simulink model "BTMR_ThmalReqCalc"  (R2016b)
settings: Solver=FixedStepDiscrete  StartTime=0.0  StopTime=10.0  FixedStep=0.1  RelTol=1e-3  EnableMultiTasking=on
undefined symbols (not defined in the file or in its folder): BMS_cntThmStbNum_C, BTMR_cntThmalReqVal_C, BTMR_flgCoolPwrCal_C, BTMR_pChrgClntPwrLv1_C, BTMR_pChrgClntPwrLv2_C, BTMR_pChrgClntPwrLv3_C, BTMR_pChrgClntPwrLv4_C, BTMR_pChrgClntPwrLv5_C, BTMR_pChrgClntPwrLv6_C, BTMR_pCoolPwrVal_C, BTMR_pHtgACPwrReq_C, BTMR_pHtgDCPwrReq_C, BTMR_pHtgDrvPwrReq_C, BTMR_pHtgsStage1_CUR, BTMR_pHtgsStage2_CUR, BTMR_pNormClntPwrLv1_C, BTMR_pNormClntPwrLv2_C, BTMR_pNormClntPwrLv3_C, BTMR_r861BrsDrvSoc_C, BTMR_r861HtgDrvSoc_C, BTMR_r891BrsDrvSoc_C, BTMR_r891HtgDrvSoc_C, BTMR_rCoolClbFlg_C, BTMR_rFlashClbFlg_C, BTMR_rHeatClbFlg_C, BTMR_t861BrsDiffLv0Temp_C, BTMR_t861BrsDiffLv1Temp_C, BTMR_t861CoolChrgAces2Temp_C, BTMR_t861CoolChrgAces3Temp_C, BTMR_t861CoolChrgAcesTemp_C, BTMR_t861CoolChrgDiffDebTemp_C, BTMR_t861CoolChrgEndDiffTemp_C, BTMR_t861CoolChrgExitLv2Temp_C, BTMR_t861CoolChrgExitLv3Temp_C, BTMR_t861CoolChrgExitTemp_C, BTMR_t861CoolChrgIntLv0Temp_C, BTMR_t861CoolChrgIntLv1Temp_C, BTMR_t861CoolChrgIntLv2Temp_C, BTMR_t861CoolChrgIntLv3Temp_C, BTMR_t861CoolChrgIntLv4Temp_C, BTMR_t861CoolChrgIntLv5Temp_C, BTMR_t861CoolDCDebTemp_C, BTMR_t861CoolNormAcesTemp_C, BTMR_t861CoolNormDiffDebTemp_C, BTMR_t861CoolNormEndDiffTemp_C, BTMR_t861CoolNormExitLv2Temp_C, BTMR_t861CoolNormExitLv3Temp_C, BTMR_t861CoolNormExitTemp_C, BTMR_t861CoolNormIntLv0Temp_C, BTMR_t861CoolNormIntLv1Temp_C, BTMR_t861CoolNormLv2Temp_C, BTMR_t861CoolNormLv3Temp_C, BTMR_t861HtgACDiffDebTemp_C, BTMR_t861HtgACEndDiffTemp_C, BTMR_t861HtgACStartHiTemp_C, BTMR_t861HtgACStartLoTemp_C, BTMR_t861HtgACStopTemp_C, BTMR_t861HtgDCDiffDebTemp_C, BTMR_t861HtgDCEndDiffTemp_C, BTMR_t861HtgDCIntLv0Temp_C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
libraries: AIWAYS_Powertrain_BMS_lib x78, simulink x9
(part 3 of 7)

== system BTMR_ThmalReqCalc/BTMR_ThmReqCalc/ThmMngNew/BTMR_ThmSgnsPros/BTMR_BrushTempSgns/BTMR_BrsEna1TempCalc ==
  BSPR_tCellTempMin : Inport
  BSPR_tCellTempMax : Inport  Port=2
  BMSDebounceStartZero : AIWAYS_Powertrain_BMS_lib/Debounce & Delay/BMSDebounceStartZero
  Constant1 : Constant  Value=BTMR_tiTempBase_C
  Constant13 : Constant  Value=BTMR_t891CoolChrgAcesTemp_C
  Constant17 : Constant  Value=BTMR_t891HtgDCStartHiTemp_C
  Constant2 : Constant  Value=BTMR_tiTempDebs_C
  Logical Operator2 : Logic  AllPortsSameDT=off  OutDataTypeStr=boolean
  Relational Operator8 : RelationalOperator  OutDataTypeStr=boolean  RndMeth=Simplest
  Relational Operator9 : RelationalOperator  Operator=<  OutDataTypeStr=boolean  RndMeth=Simplest
  BTMR_flgBrsEna1Temp : Outport
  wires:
  Relational Operator8/1 -> Logical Operator2/1
  Relational Operator9/1 -> Logical Operator2/2
  Constant13/1 -> Relational Operator9/2
  Constant17/1 -> Relational Operator8/2
  BSPR_tCellTempMin/1 -> Relational Operator8/1
  BSPR_tCellTempMax/1 -> Relational Operator9/1
  Logical Operator2/1 -> BMSDebounceStartZero/1
  BMSDebounceStartZero/1 -> BTMR_flgBrsEna1Temp/1
  Constant2/1 -> BMSDebounceStartZero/4, BMSDebounceStartZero/2
  Constant1/1 -> BMSDebounceStartZero/5, BMSDebounceStartZero/3

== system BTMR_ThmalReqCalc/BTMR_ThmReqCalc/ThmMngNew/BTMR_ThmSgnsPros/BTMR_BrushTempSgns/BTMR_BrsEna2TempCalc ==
  BSPR_tCellTempMin : Inport
  BSPR_tCellTempMax : Inport  Port=2
  BMSDebounceStartZero : AIWAYS_Powertrain_BMS_lib/Debounce & Delay/BMSDebounceStartZero
  Constant1 : Constant  Value=BTMR_tiTempBase_C
  Constant14 : Constant  Value=BTMR_t891HtgACStartHiTemp_C
  Constant16 : Constant  Value=BTMR_t891CoolNormAcesTemp_C
  Constant2 : Constant  Value=BTMR_tiTempDebs_C
  Logical Operator3 : Logic  AllPortsSameDT=off  OutDataTypeStr=boolean
  Relational Operator10 : RelationalOperator  OutDataTypeStr=boolean  RndMeth=Simplest
  Relational Operator11 : RelationalOperator  Operator=<  OutDataTypeStr=boolean  RndMeth=Simplest
  BTMR_flgBrsEna2Temp : Outport
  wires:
  BMSDebounceStartZero/1 -> BTMR_flgBrsEna2Temp/1
  BSPR_tCellTempMax/1 -> Relational Operator11/1
  BSPR_tCellTempMin/1 -> Relational Operator10/1
  Logical Operator3/1 -> BMSDebounceStartZero/1
  Relational Operator10/1 -> Logical Operator3/1
  Relational Operator11/1 -> Logical Operator3/2
  Constant14/1 -> Relational Operator10/2
  Constant16/1 -> Relational Operator11/2
  Constant2/1 -> BMSDebounceStartZero/4, BMSDebounceStartZero/2
  Constant1/1 -> BMSDebounceStartZero/5, BMSDebounceStartZero/3

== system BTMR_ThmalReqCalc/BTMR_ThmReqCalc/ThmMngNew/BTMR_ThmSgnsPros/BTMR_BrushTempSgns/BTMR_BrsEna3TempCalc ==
  BSPR_tCellTempMin : Inport
  BSPR_tCellTempMax : Inport  Port=2
  BMSDebounceStartZero : AIWAYS_Powertrain_BMS_lib/Debounce & Delay/BMSDebounceStartZero
  Constant1 : Constant  Value=BTMR_tiTempBase_C
  Constant19 : Constant  Value=BTMR_t891CoolNormAcesTemp_C
  Constant2 : Constant  Value=BTMR_tiTempDebs_C
  Constant20 : Constant  Value=BTMR_t891HtgDrvStartHiTemp_C
  Logical Operator4 : Logic  AllPortsSameDT=off  OutDataTypeStr=boolean
  Relational Operator12 : RelationalOperator  Operator=>  OutDataTypeStr=boolean  RndMeth=Simplest
  Relational Operator13 : RelationalOperator  Operator=<  OutDataTypeStr=boolean  RndMeth=Simplest
  BTMR_flgBrsEna3Temp : Outport
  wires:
  BSPR_tCellTempMax/1 -> Relational Operator13/1
  BMSDebounceStartZero/1 -> BTMR_flgBrsEna3Temp/1
  Relational Operator12/1 -> Logical Operator4/1
  Constant19/1 -> Relational Operator13/2
  Relational Operator13/1 -> Logical Operator4/2
  Constant20/1 -> Relational Operator12/2
  Logical Operator4/1 -> BMSDebounceStartZero/1
  BSPR_tCellTempMin/1 -> Relational Operator12/1
  Constant2/1 -> BMSDebounceStartZero/4, BMSDebounceStartZero/2
  Constant1/1 -> BMSDebounceStartZero/5, BMSDebounceStartZero/3

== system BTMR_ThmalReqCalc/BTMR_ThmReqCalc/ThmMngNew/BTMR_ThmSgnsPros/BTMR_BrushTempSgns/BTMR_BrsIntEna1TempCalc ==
  BSPR_tClntUsT : Inport
  BMSDebounceStartZero : AIWAYS_Powertrain_BMS_lib/Debounce & Delay/BMSDebounceStartZero
  Constant1 : Constant  Value=BTMR_tiTempBase_C
  Constant13 : Constant  Value=BTMR_t891CoolChrgAcesTemp_C
  Constant17 : Constant  Value=BTMR_t891HtgDCStartHiTemp_C
  Constant2 : Constant  Value=BTMR_tiTempDebs_C
  Logical Operator2 : Logic  AllPortsSameDT=off  OutDataTypeStr=boolean
  Relational Operator8 : RelationalOperator  OutDataTypeStr=boolean  RndMeth=Simplest
  Relational Operator9 : RelationalOperator  Operator=<  OutDataTypeStr=boolean  RndMeth=Simplest
  BTMR_flgBrsIntEna1Temp : Outport
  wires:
  BMSDebounceStartZero/1 -> BTMR_flgBrsIntEna1Temp/1
  Logical Operator2/1 -> BMSDebounceStartZero/1
  BSPR_tClntUsT/1 -> Relational Operator9/1, Relational Operator8/1
  Constant17/1 -> Relational Operator8/2
  Constant13/1 -> Relational Operator9/2
  Relational Operator9/1 -> Logical Operator2/2
  Relational Operator8/1 -> Logical Operator2/1
  Constant2/1 -> BMSDebounceStartZero/4, BMSDebounceStartZero/2
  Constant1/1 -> BMSDebounceStartZero/5, BMSDebounceStartZero/3

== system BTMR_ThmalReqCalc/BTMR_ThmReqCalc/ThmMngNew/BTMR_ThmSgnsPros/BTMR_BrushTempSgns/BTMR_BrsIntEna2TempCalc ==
  BSPR_tClntUsT : Inport
  BMSDebounceStartZero : AIWAYS_Powertrain_BMS_lib/Debounce & Delay/BMSDebounceStartZero
  Constant1 : Constant  Value=BTMR_tiTempBase_C
  Constant14 : Constant  Value=BTMR_t891HtgACStartHiTemp_C
  Constant16 : Constant  Value=BTMR_t891CoolNormAcesTemp_C
  Constant2 : Constant  Value=BTMR_tiTempDebs_C
  Logical Operator3 : Logic  AllPortsSameDT=off  OutDataTypeStr=boolean
  Relational Operator10 : RelationalOperator  OutDataTypeStr=boolean  RndMeth=Simplest
  Relational Operator11 : RelationalOperator  Operator=<  OutDataTypeStr=boolean  RndMeth=Simplest
  BTMR_flgBrsIntEna2Temp : Outport
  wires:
  Constant16/1 -> Relational Operator11/2
  Constant14/1 -> Relational Operator10/2
  Relational Operator11/1 -> Logical Operator3/2
  Relational Operator10/1 -> Logical Operator3/1
  Logical Operator3/1 -> BMSDebounceStartZero/1
  BSPR_tClntUsT/1 -> Relational Operator11/1, Relational Operator10/1
  BMSDebounceStartZero/1 -> BTMR_flgBrsIntEna2Temp/1
  Constant2/1 -> BMSDebounceStartZero/4, BMSDebounceStartZero/2
  Constant1/1 -> BMSDebounceStartZero/5, BMSDebounceStartZero/3

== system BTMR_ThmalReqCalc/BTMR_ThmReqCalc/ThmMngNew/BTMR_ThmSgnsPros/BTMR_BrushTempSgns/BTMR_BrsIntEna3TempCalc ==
  BSPR_tClntUsT : Inport
  BMSDebounceStartZero : AIWAYS_Powertrain_BMS_lib/Debounce & Delay/BMSDebounceStartZero
  Constant1 : Constant  Value=BTMR_tiTempBase_C
  Constant19 : Constant  Value=BTMR_t891CoolNormAcesTemp_C
  Constant2 : Constant  Value=BTMR_tiTempDebs_C
  Constant20 : Constant  Value=BTMR_t891HtgDrvStartHiTemp_C
  Logical Operator4 : Logic  AllPortsSameDT=off  OutDataTypeStr=boolean
  Relational Operator12 : RelationalOperator  Operator=>  OutDataTypeStr=boolean  RndMeth=Simplest
  Relational Operator13 : RelationalOperator  Operator=<  OutDataTypeStr=boolean  RndMeth=Simplest
  BTMR_flgBrsIntEna3Temp : Outport
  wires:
  Logical Operator4/1 -> BMSDebounceStartZero/1
  Constant20/1 -> Relational Operator12/2
  Relational Operator13/1 -> Logical Operator4/2
  Constant19/1 -> Relational Operator13/2
  Relational Operator12/1 -> Logical Operator4/1
  BMSDebounceStartZero/1 -> BTMR_flgBrsIntEna3Temp/1
  BSPR_tClntUsT/1 -> Relational Operator13/1, Relational Operator12/1
  Constant2/1 -> BMSDebounceStartZero/4, BMSDebounceStartZero/2
  Constant1/1 -> BMSDebounceStartZero/5, BMSDebounceStartZero/3

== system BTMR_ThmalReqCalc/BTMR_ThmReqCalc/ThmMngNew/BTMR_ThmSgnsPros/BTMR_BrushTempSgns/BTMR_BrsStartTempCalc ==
  BSPR_tCellTempMin : Inport
  BSPR_tCellTempMax : Inport  Port=2
  Add : Sum  Inputs=+-
  BMSDebounceStartZero : AIWAYS_Powertrain_BMS_lib/Debounce & Delay/BMSDebounceStartZero
  Constant1 : Constant  Value=BTMR_tiTempBase_C
  Constant2 : Constant  Value=BTMR_t891BrsDiffLv1Temp_C
  Constant3 : Constant  Value=BTMR_tiTempDebs_C
  Constant4 : Constant  Value=BTMR_tBrsMinCellTempThre_C
  Logical Operator4 : Logic  AllPortsSameDT=off  OutDataTypeStr=boolean
  Relational Operator2 : RelationalOperator  OutDataTypeStr=boolean  RndMeth=Simplest
  Relational Operator4 : RelationalOperator  OutDataTypeStr=boolean  RndMeth=Simplest
  BTMR_flgBrsStartTemp : Outport
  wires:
  BMSDebounceStartZero/1 -> BTMR_flgBrsStartTemp/1
  Add/1 -> Relational Operator2/1
  Constant2/1 -> Relational Operator2/2
  Relational Operator2/1 -> Logical Operator4/1
  BSPR_tCellTempMax/1 -> Add/1
  Constant3/1 -> BMSDebounceStartZero/4, BMSDebounceStartZero/2
  Constant1/1 -> BMSDebounceStartZero/5, BMSDebounceStartZero/3
  BSPR_tCellTempMin/1 -> Relational Operator4/1, Add/2
  Constant4/1 -> Relational Operator4/2
  Relational Operator4/1 -> Logical Operator4/2
  Logical Operator4/1 -> BMSDebounceStartZero/1

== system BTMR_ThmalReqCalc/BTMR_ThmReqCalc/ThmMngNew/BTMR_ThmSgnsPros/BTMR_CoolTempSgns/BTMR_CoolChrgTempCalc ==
  BSPR_tCellTempMax : Inport
  BTMR_CoolChrgDnaTempCalc : Subsystem
  BTMR_CoolChrgStage2EnaTempCalc : Subsystem
  BTMR_CoolChrgStage2ExtTempCalc : Subsystem
  BTMR_CoolChrgStage3EnaTempCalc : Subsystem
  BTMR_CoolChrgStage3ExtTempCalc : Subsystem
  Bus Creator : BusCreator  Inputs=5
  BTMR_flgCoolChrgTempSgns : Outport
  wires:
  BTMR_CoolChrgStage2EnaTempCalc/1(BTMR_flgCoolChrgStage2EnaTemp) -> Bus Creator/2  "BTMR_flgCoolChrgStage2EnaTemp"
  BTMR_CoolChrgStage3EnaTempCalc/1(BTMR_flgCoolChrgStage3EnaTemp) -> Bus Creator/3  "BTMR_flgCoolChrgStage3EnaTemp"
  BTMR_CoolChrgStage3ExtTempCalc/1(BTMR_flgCoolChrgStage3ExtTemp) -> Bus Creator/5  "BTMR_flgCoolChrgStage3ExtTemp"
  BTMR_CoolChrgStage2ExtTempCalc/1(BTMR_flgCoolChrgStage2ExtTemp) -> Bus Creator/4  "BTMR_flgCoolChrgStage2ExtTemp"
  BSPR_tCellTempMax/1 -> BTMR_CoolChrgStage3ExtTempCalc/1(BSPR_tCellTempMax), BTMR_CoolChrgStage2ExtTempCalc/1(BSPR_tCellTempMax), BTMR_CoolChrgDnaTempCalc/1(BSPR_tCellTempMax), BTMR_CoolChrgStage2EnaTempCalc/1(BSPR_tCellTempMax), BTMR_CoolChrgStage3EnaTempCalc/1(BSPR_tCellTempMax)
  BTMR_CoolChrgDnaTempCalc/1(BTMR_flgCoolChrgDnaTemp) -> Bus Creator/1  "BTMR_flgCoolChrgDnaTemp"
  Bus Creator/1 -> BTMR_flgCoolChrgTempSgns/1  "BTMR_flgCoolChrgTempSgns"

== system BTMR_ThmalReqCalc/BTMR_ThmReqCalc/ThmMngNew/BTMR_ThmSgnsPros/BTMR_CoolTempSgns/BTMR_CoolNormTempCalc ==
  BSPR_tCellTempMax : Inport
  BTMR_CoolNormDnaTempCalc : Subsystem
  BTMR_CoolNormStage2EnaTempCalc : Subsystem
  BTMR_CoolNormStage2ExtTempCalc : Subsystem
  BTMR_CoolNormStage3EnaTempCalc : Subsystem
  BTMR_CoolNormStage3ExtTempCalc : Subsystem
  Bus Creator : BusCreator  Inputs=5
  BTMR_flgCoolNormTempSgns : Outport
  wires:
  BTMR_CoolNormDnaTempCalc/1(BTMR_flgCoolNormDnaTemp) -> Bus Creator/1  "BTMR_flgCoolNormDnaTemp"
  BTMR_CoolNormStage2EnaTempCalc/1(BTMR_flgCoolNormStage2EnaTemp) -> Bus Creator/2  "BTMR_flgCoolNormStage2EnaTemp"
  BTMR_CoolNormStage3EnaTempCalc/1(BTMR_flgCoolNormStage3EnaTemp) -> Bus Creator/3  "BTMR_flgCoolNormStage3EnaTemp"
  BTMR_CoolNormStage3ExtTempCalc/1(BTMR_flgCoolNormStage3ExtTemp) -> Bus Creator/5  "BTMR_flgCoolNormStage3ExtTemp"
  BTMR_CoolNormStage2ExtTempCalc/1(BTMR_flgCoolNormStage2ExtTemp) -> Bus Creator/4  "BTMR_flgCoolNormStage2ExtTemp"
  BSPR_tCellTempMax/1 -> BTMR_CoolNormDnaTempCalc/1(BSPR_tCellTempMax), BTMR_CoolNormStage2EnaTempCalc/1(BSPR_tCellTempMax), BTMR_CoolNormStage3ExtTempCalc/1(BSPR_tCellTempMax), BTMR_CoolNormStage2ExtTempCalc/1(BSPR_tCellTempMax), BTMR_CoolNormStage3EnaTempCalc/1(BSPR_tCellTempMax)
  Bus Creator/1 -> BTMR_flgCoolNormTempSgns/1  "BTMR_flgCoolNormTempSgns"

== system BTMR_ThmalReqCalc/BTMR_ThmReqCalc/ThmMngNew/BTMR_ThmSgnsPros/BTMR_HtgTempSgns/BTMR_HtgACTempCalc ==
  BSPR_tCellTempMin : Inport
  BSPR_tCellTempMax : Inport  Port=2
  BTMR_HtgACDnaTempCalc : Subsystem
  Bus Creator : BusCreator  Inputs=1
  BTMR_flgHtgACTempSgns : Outport
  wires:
  BTMR_HtgACDnaTempCalc/1(BTMR_flgHtgACDnaTemp) -> Bus Creator/1  "BTMR_flgHtgACDnaTemp"
  BSPR_tCellTempMin/1 -> BTMR_HtgACDnaTempCalc/1(BSPR_tCellTempMin)
  Bus Creator/1 -> BTMR_flgHtgACTempSgns/1  "BTMR_flgHtgACTempSgns"
  BSPR_tCellTempMax/1 -> BTMR_HtgACDnaTempCalc/2(BSPR_tCellTempMax)

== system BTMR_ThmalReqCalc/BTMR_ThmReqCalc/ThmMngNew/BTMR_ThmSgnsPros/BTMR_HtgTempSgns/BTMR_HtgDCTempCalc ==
  BSPR_tCellTempMin : Inport
  BSPR_tCellTempMax : Inport  Port=2
  BTMR_HtgDCDnaTempCalc : Subsystem
  BTMR_HtgDCStage2EnaTempCalc : Subsystem
  Bus Creator : BusCreator  Inputs=2
  BTMR_flgHtgDCTempSgns : Outport
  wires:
  BSPR_tCellTempMax/1 -> BTMR_HtgDCDnaTempCalc/2(BSPR_tCellTempMax), BTMR_HtgDCStage2EnaTempCalc/2(BSPR_tCellTempMax)
  BTMR_HtgDCDnaTempCalc/1(BTMR_flgHtgDCDnaTemp) -> Bus Creator/2  "BTMR_flgHtgDCDnaTemp"
  BTMR_HtgDCStage2EnaTempCalc/1(BTMR_flgHtgDCStage2EnaTemp) -> Bus Creator/1  "BTMR_flgHtgDCStage2EnaTemp"
  BSPR_tCellTempMin/1 -> BTMR_HtgDCDnaTempCalc/1(BSPR_tCellTempMin), BTMR_HtgDCStage2EnaTempCalc/1(BSPR_tCellTempMin)
  Bus Creator/1 -> BTMR_flgHtgDCTempSgns/1  "BTMR_flgHtgDCTempSgns"

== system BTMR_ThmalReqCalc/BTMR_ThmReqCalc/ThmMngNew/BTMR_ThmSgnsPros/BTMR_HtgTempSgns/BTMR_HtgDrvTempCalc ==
  BSPR_tCellTempMin : Inport
  BSPR_tCellTempMax : Inport  Port=2
  BTMR_HtgDrvDnaTempCalc : Subsystem
  Bus Creator : BusCreator  Inputs=1
  BTMR_flgHtgDrvTempSgns : Outport
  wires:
  BTMR_HtgDrvDnaTempCalc/1(BTMR_flgHtgDrvDnaTemp) -> Bus Creator/1  "BTMR_flgHtgDrvDnaTemp"
  BSPR_tCellTempMin/1 -> BTMR_HtgDrvDnaTempCalc/1(BSPR_tCellTempMin)
  Bus Creator/1 -> BTMR_flgHtgDrvTempSgns/1  "BTMR_flgHtgDrvTempSgns"
  BSPR_tCellTempMax/1 -> BTMR_HtgDrvDnaTempCalc/2(BSPR_tCellTempMax)

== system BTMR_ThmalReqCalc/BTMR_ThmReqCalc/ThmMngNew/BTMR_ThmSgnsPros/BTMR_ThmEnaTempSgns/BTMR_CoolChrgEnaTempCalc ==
  BSPR_tCellTempMin : Inport
  BSPR_tCellTempMax : Inport  Port=2
  Add : Sum
  Add1 : Sum  Inputs=+-
  Add2 : Sum  Inputs=+-
  BMSDebounceStartZero : AIWAYS_Powertrain_BMS_lib/Debounce & Delay/BMSDebounceStartZero
  Constant1 : Constant  Value=BTMR_tiTempBase_C
  Constant2 : Constant  Value=BTMR_tiTempDebs_C
  Constant27 : Constant  Value=BTMR_t891CoolChrgAcesTemp_C
  Constant3 : Constant  Value=BTMR_t891HtgDCStopMinTemp_C
  Constant4 : Constant  Value=BTMR_t891CoolDCDebTemp_C
  Constant5 : Constant  Value=BTMR_t891CoolChrgDiffDebTemp_C
  Constant6 : Constant  Value=BTMR_t891CoolChrgEndDiffTemp_C
  Logical Operator : Logic  Inputs=3  AllPortsSameDT=off  OutDataTypeStr=boolean
  Relational Operator1 : RelationalOperator  OutDataTypeStr=boolean  RndMeth=Simplest
  Relational Operator19 : RelationalOperator  OutDataTypeStr=boolean  RndMeth=Simplest
  Relational Operator2 : RelationalOperator  Operator=<  OutDataTypeStr=boolean  RndMeth=Simplest
  BTMR_flgCoolChrgEnaTemp : Outport
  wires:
  Logical Operator/1 -> BMSDebounceStartZero/1
  Constant27/1 -> Relational Operator19/2
  BMSDebounceStartZero/1 -> BTMR_flgCoolChrgEnaTemp/1
  Constant2/1 -> BMSDebounceStartZero/4, BMSDebounceStartZero/2
  Constant1/1 -> BMSDebounceStartZero/5, BMSDebounceStartZero/3
  Add1/1 -> Relational Operator2/1
  Relational Operator1/1 -> Logical Operator/3
  Add2/1 -> Relational Operator2/2
  Add/1 -> Relational Operator1/2
  Constant5/1 -> Add2/2
  BSPR_tCellTempMax/1 -> Add1/1, Relational Operator19/1
  BSPR_tCellTempMin/1 -> Relational Operator1/1, Add1/2
  Relational Operator2/1 -> Logical Operator/2
  Constant4/1 -> Add/2
  Constant3/1 -> Add/1
  Constant6/1 -> Add2/1
  Relational Operator19/1 -> Logical Operator/1

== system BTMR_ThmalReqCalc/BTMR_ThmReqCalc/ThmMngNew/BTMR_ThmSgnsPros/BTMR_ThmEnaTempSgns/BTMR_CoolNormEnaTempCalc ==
  BSPR_tCellTempMin : Inport
  BSPR_tCellTempMax : Inport  Port=2
  Add1 : Sum  Inputs=+-
  Add2 : Sum  Inputs=+-
  BMSDebounceStartZero : AIWAYS_Powertrain_BMS_lib/Debounce & Delay/BMSDebounceStartZero
  Constant1 : Constant  Value=BTMR_tiTempBase_C
  Constant2 : Constant  Value=BTMR_tiTempDebs_C
  Constant28 : Constant  Value=BTMR_t891CoolNormAcesTemp_C
  Constant3 : Constant  Value=BTMR_t891CoolNormDiffDebTemp_C
  Constant4 : Constant  Value=BTMR_t891CoolNormEndDiffTemp_C
  Logical Operator : Logic  AllPortsSameDT=off  OutDataTypeStr=boolean
  Relational Operator2 : RelationalOperator  Operator=<  OutDataTypeStr=boolean  RndMeth=Simplest
  Relational Operator20 : RelationalOperator  OutDataTypeStr=boolean  RndMeth=Simplest
  BTMR_flgCoolNormEnaTemp : Outport
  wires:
  Logical Operator/1 -> BMSDebounceStartZero/1
  BMSDebounceStartZero/1 -> BTMR_flgCoolNormEnaTemp/1
  Constant28/1 -> Relational Operator20/2
  Constant2/1 -> BMSDebounceStartZero/4, BMSDebounceStartZero/2
  Constant1/1 -> BMSDebounceStartZero/5, BMSDebounceStartZero/3
  Add2/1 -> Relational Operator2/2
  BSPR_tCellTempMin/1 -> Add1/2
  Constant3/1 -> Add2/2
  Add1/1 -> Relational Operator2/1
  Constant4/1 -> Add2/1
  BSPR_tCellTempMax/1 -> Add1/1, Relational Operator20/1
  Relational Operator20/1 -> Logical Operator/1
  Relational Operator2/1 -> Logical Operator/2

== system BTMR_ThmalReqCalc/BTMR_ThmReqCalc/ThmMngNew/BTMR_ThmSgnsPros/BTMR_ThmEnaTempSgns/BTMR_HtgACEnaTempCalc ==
  BSPR_tCellTempMin : Inport
  BSPR_tCellTempMax : Inport  Port=2
  BMSDebounceStartZero : AIWAYS_Powertrain_BMS_lib/Debounce & Delay/BMSDebounceStartZero
  Constant1 : Constant  Value=BTMR_tiTempBase_C
  Constant2 : Constant  Value=BTMR_tiTempDebs_C
  Constant23 : Constant  Value=BTMR_t891HtgACStartLoTemp_C
  Constant24 : Constant  Value=BTMR_t891HtgACStartHiTemp_C
  Constant3 : Constant  Value=BTMR_t891HtgACDiffDebTemp_C
  Constant4 : Constant  Value=BTMR_t891HtgACEndDiffTemp_C
  Logical Operator6 : Logic  Inputs=3  AllPortsSameDT=off  OutDataTypeStr=boolean
  Relational Operator1 : RelationalOperator  Operator=<  OutDataTypeStr=boolean  RndMeth=Simplest
  Relational Operator14 : RelationalOperator  OutDataTypeStr=boolean  RndMeth=Simplest
  Relational Operator15 : RelationalOperator  Operator=<  OutDataTypeStr=boolean  RndMeth=Simplest
  Sum1 : Sum  Inputs=+-  OutDataTypeStr=Inherit: Inherit via back propagation  RndMeth=Zero
  Sum2 : Sum  Inputs=+-  OutDataTypeStr=Inherit: Inherit via back propagation  RndMeth=Zero
  BTMR_flgHtgACEnaTemp : Outport
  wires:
  BMSDebounceStartZero/1 -> BTMR_flgHtgACEnaTemp/1
  Relational Operator14/1 -> Logical Operator6/2
  Constant24/1 -> Relational Operator15/2
  Constant23/1 -> Relational Operator14/2
  Relational Operator15/1 -> Logical Operator6/3
  Logical Operator6/1 -> BMSDebounceStartZero/1
  Constant2/1 -> BMSDebounceStartZero/4, BMSDebounceStartZero/2
  Constant1/1 -> BMSDebounceStartZero/5, BMSDebounceStartZero/3
  Constant3/1 -> Sum2/2
  Sum2/1 -> Relational Operator1/2
  BSPR_tCellTempMax/1 -> Sum1/1
  Relational Operator1/1 -> Logical Operator6/1
  Sum1/1 -> Relational Operator1/1
  BSPR_tCellTempMin/1 -> Sum1/2, Relational Operator15/1, Relational Operator14/1
  Constant4/1 -> Sum2/1

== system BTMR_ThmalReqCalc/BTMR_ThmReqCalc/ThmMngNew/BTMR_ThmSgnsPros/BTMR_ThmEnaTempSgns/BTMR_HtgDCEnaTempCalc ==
  BSPR_tCellTempMin : Inport
  BSPR_tCellTempMax : Inport  Port=2
  BMSDebounceStartZero : AIWAYS_Powertrain_BMS_lib/Debounce & Delay/BMSDebounceStartZero
  Constant1 : Constant  Value=BTMR_tiTempBase_C
  Constant2 : Constant  Value=BTMR_tiTempDebs_C
  Constant23 : Constant  Value=BTMR_t891HtgDCStopMaxTemp_C
  Constant25 : Constant  Value=BTMR_t891HtgDCStartHiTemp_C
  Constant26 : Constant  Value=BTMR_t891HtgDCStartLoTemp_C
  Constant3 : Constant  Value=BTMR_t891HtgDCDiffDebTemp_C
  Constant4 : Constant  Value=BTMR_t891HtgDCEndDiffTemp_C
  Constant5 : Constant  Value=BTMR_tHtgDCMaxTempDeb_C
  Logical Operator6 : Logic  Inputs=4  AllPortsSameDT=off  OutDataTypeStr=boolean
  Relational Operator1 : RelationalOperator  Operator=<  OutDataTypeStr=boolean  RndMeth=Simplest
  Relational Operator16 : RelationalOperator  Operator=>  OutDataTypeStr=boolean  RndMeth=Simplest
  Relational Operator17 : RelationalOperator  Operator=<  OutDataTypeStr=boolean  RndMeth=Simplest
  Relational Operator2 : RelationalOperator  Operator=<  OutDataTypeStr=boolean  RndMeth=Simplest
  Sum1 : Sum  Inputs=+-  OutDataTypeStr=Inherit: Inherit via back propagation  RndMeth=Zero
  Sum2 : Sum  Inputs=+-  OutDataTypeStr=Inherit: Inherit via back propagation  RndMeth=Zero
  Sum3 : Sum  Inputs=+-  OutDataTypeStr=Inherit: Inherit via back propagation  RndMeth=Zero
  BTMR_flgHtgDCEnaTemp : Outport
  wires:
  BMSDebounceStartZero/1 -> BTMR_flgHtgDCEnaTemp/1
  Constant25/1 -> Relational Operator17/2
  Relational Operator17/1 -> Logical Operator6/4
  Constant26/1 -> Relational Operator16/2
  Relational Operator16/1 -> Logical Operator6/3
  Logical Operator6/1 -> BMSDebounceStartZero/1
  Constant2/1 -> BMSDebounceStartZero/4, BMSDebounceStartZero/2
  Constant1/1 -> BMSDebounceStartZero/5, BMSDebounceStartZero/3
  Sum1/1 -> Relational Operator1/1
  BSPR_tCellTempMin/1 -> Relational Operator17/1, Relational Operator16/1, Sum1/2
  BSPR_tCellTempMax/1 -> Sum1/1, Relational Operator2/1
  Sum2/1 -> Relational Operator1/2
  Constant3/1 -> Sum2/2
  Constant4/1 -> Sum2/1
  Relational Operator1/1 -> Logical Operator6/2
  Constant23/1 -> Sum3/1
  Constant5/1 -> Sum3/2
  Sum3/1 -> Relational Operator2/2
  Relational Operator2/1 -> Logical Operator6/1

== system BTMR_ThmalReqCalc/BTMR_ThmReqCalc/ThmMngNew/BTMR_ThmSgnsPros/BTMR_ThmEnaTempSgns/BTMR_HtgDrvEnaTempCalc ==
  BSPR_tCellTempMin : Inport
  BSPR_tCellTempMax : Inport  Port=2
  BMSDebounceStartZero : AIWAYS_Powertrain_BMS_lib/Debounce & Delay/BMSDebounceStartZero
  Constant1 : Constant  Value=BTMR_tiTempBase_C
  Constant2 : Constant  Value=BTMR_tiTempDebs_C
  Constant21 : Constant  Value=BTMR_t891HtgDrvStartLoTemp_C
  Constant22 : Constant  Value=BTMR_t891HtgDrvStartHiTemp_C
  Constant3 : Constant  Value=BTMR_t891HtgDrvDiffDebTemp_C
  Constant4 : Constant  Value=BTMR_t891HtgDrvEndDiffTemp_C
  Logical Operator6 : Logic  Inputs=3  AllPortsSameDT=off  OutDataTypeStr=boolean
  Relational Operator1 : RelationalOperator  OutDataTypeStr=boolean  RndMeth=Simplest
  Relational Operator18 : RelationalOperator  Operator=<=  OutDataTypeStr=boolean  RndMeth=Simplest
  Relational Operator2 : RelationalOperator  Operator=<  OutDataTypeStr=boolean  RndMeth=Simplest
  Sum1 : Sum  Inputs=+-  OutDataTypeStr=Inherit: Inherit via back propagation  RndMeth=Zero
  Sum2 : Sum  Inputs=+-  OutDataTypeStr=Inherit: Inherit via back propagation  RndMeth=Zero
  BTMR_flgHtgDrvEnaTemp : Outport
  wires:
  Constant22/1 -> Relational Operator18/2
  BMSDebounceStartZero/1 -> BTMR_flgHtgDrvEnaTemp/1
  Logical Operator6/1 -> BMSDebounceStartZero/1
  Constant21/1 -> Relational Operator1/2
  Relational Operator18/1 -> Logical Operator6/2
  Relational Operator1/1 -> Logical Operator6/3
  Constant2/1 -> BMSDebounceStartZero/4, BMSDebounceStartZero/2
  Constant1/1 -> BMSDebounceStartZero/5, BMSDebounceStartZero/3
  Sum1/1 -> Relational Operator2/1
  Constant4/1 -> Sum2/1
  Sum2/1 -> Relational Operator2/2
  BSPR_tCellTempMax/1 -> Sum1/1
  Constant3/1 -> Sum2/2
  Relational Operator2/1 -> Logical Operator6/1
  BSPR_tCellTempMin/1 -> Sum1/2, Relational Operator1/1, Relational Operator18/1

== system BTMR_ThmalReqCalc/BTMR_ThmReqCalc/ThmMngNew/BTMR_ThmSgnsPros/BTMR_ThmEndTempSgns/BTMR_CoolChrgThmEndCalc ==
  BTMR_flgBMSSgns : Inport
  BSPR_tCellTempMax : Inport  Port=2
  BSPR_tCellTempMin : Inport  Port=3
  Add : Sum  Inputs=+-
  BMSDebounceStartZero : AIWAYS_Powertrain_BMS_lib/Debounce & Delay/BMSDebounceStartZero
  Bus Selector : BusSelector  OutputSignals=BTMR_flgBMSDChrg
  Constant1 : Constant  Value=BTMR_tiTempBase_C
  Constant14 : Constant  Value=BTMR_t891CoolChrgEndDiffTemp_C
  Constant2 : Constant  Value=BTMR_tiTempDebs_C
  Logical Operator1 : Logic  AllPortsSameDT=off  OutDataTypeStr=boolean
  Relational Operator3 : RelationalOperator  OutDataTypeStr=boolean  RndMeth=Simplest
  BTMR_CoolChrgThmEnd : Outport
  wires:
  BMSDebounceStartZero/1 -> Logical Operator1/2
  BSPR_tCellTempMin/1 -> Add/2
  Add/1 -> Relational Operator3/1
  Constant14/1 -> Relational Operator3/2
  BSPR_tCellTempMax/1 -> Add/1
  Relational Operator3/1 -> BMSDebounceStartZero/1
  BTMR_flgBMSSgns/1 -> Bus Selector/1
  Bus Selector/1 -> Logical Operator1/1  "<BTMR_flgBMSDChrg>"
  Logical Operator1/1 -> BTMR_CoolChrgThmEnd/1
  Constant2/1 -> BMSDebounceStartZero/4, BMSDebounceStartZero/2
  Constant1/1 -> BMSDebounceStartZero/5, BMSDebounceStartZero/3

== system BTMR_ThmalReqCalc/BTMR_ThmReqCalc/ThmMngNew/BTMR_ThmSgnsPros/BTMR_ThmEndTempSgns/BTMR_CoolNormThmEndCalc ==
  BTMR_flgBMSSgns : Inport
  BSPR_tCellTempMax : Inport  Port=2
  BSPR_tCellTempMin : Inport  Port=3
  Add : Sum  Inputs=+-
  BMSDebounceStartZero : AIWAYS_Powertrain_BMS_lib/Debounce & Delay/BMSDebounceStartZero
  Bus Selector : BusSelector  OutputSignals=BTMR_flgBMSAChrg,BTMR_flgBMSDrv
  Constant1 : Constant  Value=BTMR_tiTempBase_C
  Constant14 : Constant  Value=BTMR_t891CoolNormEndDiffTemp_C
  Constant2 : Constant  Value=BTMR_tiTempDebs_C
  Logical Operator1 : Logic  AllPortsSameDT=off  OutDataTypeStr=boolean
  Logical Operator2 : Logic  Operator=OR  AllPortsSameDT=off  OutDataTypeStr=boolean
  Relational Operator3 : RelationalOperator  OutDataTypeStr=boolean  RndMeth=Simplest
  BTMR_CoolNormThmEnd : Outport
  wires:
  BTMR_flgBMSSgns/1 -> Bus Selector/1
  Relational Operator3/1 -> BMSDebounceStartZero/1
  BSPR_tCellTempMax/1 -> Add/1
  Constant14/1 -> Relational Operator3/2
  Add/1 -> Relational Operator3/1
  BSPR_tCellTempMin/1 -> Add/2
  BMSDebounceStartZero/1 -> Logical Operator1/2
  Bus Selector/1 -> Logical Operator2/1  "<BTMR_flgBMSAChrg>"
  Bus Selector/2 -> Logical Operator2/2  "<BTMR_flgBMSDrv>"
  Logical Operator2/1 -> Logical Operator1/1
  Logical Operator1/1 -> BTMR_CoolNormThmEnd/1
  Constant2/1 -> BMSDebounceStartZero/4, BMSDebounceStartZero/2
  Constant1/1 -> BMSDebounceStartZero/5, BMSDebounceStartZero/3

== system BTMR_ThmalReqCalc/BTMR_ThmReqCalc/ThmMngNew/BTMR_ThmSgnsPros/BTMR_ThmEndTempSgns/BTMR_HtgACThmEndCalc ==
  BTMR_flgBMSSgns : Inport
  BSPR_tCellTempMax : Inport  Port=2
  BSPR_tCellTempMin : Inport  Port=3
  BCMR_bAcChrgHeatFbd : Inport  Port=4
  Add : Sum  Inputs=+-
  BMSDebounceStartZero : AIWAYS_Powertrain_BMS_lib/Debounce & Delay/BMSDebounceStartZero
  Bus Selector : BusSelector  OutputSignals=BTMR_flgBMSAChrg
  Constant1 : Constant  Value=BTMR_tiTempBase_C
  Constant14 : Constant  Value=BTMR_t891HtgACEndDiffTemp_C
  Constant2 : Constant  Value=BTMR_tiTempDebs_C
  Logical Operator1 : Logic  AllPortsSameDT=off  OutDataTypeStr=boolean
  Logical Operator2 : Logic  Operator=OR  AllPortsSameDT=off  OutDataTypeStr=boolean
  Relational Operator3 : RelationalOperator  OutDataTypeStr=boolean  RndMeth=Simplest
  BTMR_HtgACThmEnd : Outport
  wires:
  Logical Operator1/1 -> BTMR_HtgACThmEnd/1
  BSPR_tCellTempMin/1 -> Add/2
  Add/1 -> Relational Operator3/1
  Constant14/1 -> Relational Operator3/2
  BSPR_tCellTempMax/1 -> Add/1
  Relational Operator3/1 -> BMSDebounceStartZero/1
  BTMR_flgBMSSgns/1 -> Bus Selector/1
  Bus Selector/1 -> Logical Operator1/1  "<BTMR_flgBMSAChrg>"
  BMSDebounceStartZero/1 -> Logical Operator2/1
  BCMR_bAcChrgHeatFbd/1 -> Logical Operator2/2
  Logical Operator2/1 -> Logical Operator1/2
  Constant2/1 -> BMSDebounceStartZero/4, BMSDebounceStartZero/2
  Constant1/1 -> BMSDebounceStartZero/5, BMSDebounceStartZero/3

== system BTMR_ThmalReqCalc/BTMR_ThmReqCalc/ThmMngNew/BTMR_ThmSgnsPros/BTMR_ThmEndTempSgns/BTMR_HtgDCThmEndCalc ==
  BTMR_flgBMSSgns : Inport
  BSPR_tCellTempMax : Inport  Port=2
  BSPR_tCellTempMin : Inport  Port=3
  Add : Sum  Inputs=+-
  BMSDebounceStartZero : AIWAYS_Powertrain_BMS_lib/Debounce & Delay/BMSDebounceStartZero
  Bus Selector : BusSelector  OutputSignals=BTMR_flgBMSDChrg
  Constant1 : Constant  Value=BTMR_tiTempBase_C
  Constant14 : Constant  Value=BTMR_t891HtgDCEndDiffTemp_C
  Constant2 : Constant  Value=BTMR_tiTempDebs_C
  Logical Operator1 : Logic  AllPortsSameDT=off  OutDataTypeStr=boolean
  Relational Operator3 : RelationalOperator  OutDataTypeStr=boolean  RndMeth=Simplest
  BTMR_HtgDCThmEnd : Outport
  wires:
  Bus Selector/1 -> Logical Operator1/1  "<BTMR_flgBMSDChrg>"
  BTMR_flgBMSSgns/1 -> Bus Selector/1
  Relational Operator3/1 -> BMSDebounceStartZero/1
  BSPR_tCellTempMax/1 -> Add/1
  Constant14/1 -> Relational Operator3/2
  Add/1 -> Relational Operator3/1
  BSPR_tCellTempMin/1 -> Add/2
  Logical Operator1/1 -> BTMR_HtgDCThmEnd/1
  BMSDebounceStartZero/1 -> Logical Operator1/2
  Constant2/1 -> BMSDebounceStartZero/4, BMSDebounceStartZero/2
  Constant1/1 -> BMSDebounceStartZero/5, BMSDebounceStartZero/3

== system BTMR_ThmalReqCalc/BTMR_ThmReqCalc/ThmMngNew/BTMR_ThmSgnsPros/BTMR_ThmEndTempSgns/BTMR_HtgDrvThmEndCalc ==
  BTMR_flgBMSSgns : Inport
  BSPR_tCellTempMax : Inport  Port=2
  BSPR_tCellTempMin : Inport  Port=3
  Add : Sum  Inputs=+-
  BMSDebounceStartZero : AIWAYS_Powertrain_BMS_lib/Debounce & Delay/BMSDebounceStartZero
  Bus Selector : BusSelector  OutputSignals=BTMR_flgBMSDrv
  Constant1 : Constant  Value=BTMR_tiTempBase_C
  Constant14 : Constant  Value=BTMR_t891HtgDrvEndDiffTemp_C
  Constant2 : Constant  Value=BTMR_tiTempDebs_C
  Logical Operator1 : Logic  AllPortsSameDT=off  OutDataTypeStr=boolean
  Relational Operator3 : RelationalOperator  OutDataTypeStr=boolean  RndMeth=Simplest
  BTMR_HtgDrvThmEnd : Outport
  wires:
  BMSDebounceStartZero/1 -> Logical Operator1/2
  Logical Operator1/1 -> BTMR_HtgDrvThmEnd/1
  BSPR_tCellTempMin/1 -> Add/2
  Add/1 -> Relational Operator3/1
  Constant14/1 -> Relational Operator3/2
  BSPR_tCellTempMax/1 -> Add/1
  Relational Operator3/1 -> BMSDebounceStartZero/1
  BTMR_flgBMSSgns/1 -> Bus Selector/1
  Bus Selector/1 -> Logical Operator1/1  "<BTMR_flgBMSDrv>"
  Constant2/1 -> BMSDebounceStartZero/4, BMSDebounceStartZero/2
  Constant1/1 -> BMSDebounceStartZero/5, BMSDebounceStartZero/3

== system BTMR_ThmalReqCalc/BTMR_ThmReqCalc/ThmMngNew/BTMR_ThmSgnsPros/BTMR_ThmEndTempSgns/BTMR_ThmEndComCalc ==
  BMCR_stBmsModeCtrl : Inport
  DSMR_stFaultRank : Inport  Port=2
  COMR_bLeadAcidChgHvOn : Inport  Port=3
  Constant13 : Constant  Value=enmBmsFaultLvl.FaultLv3  OutDataTypeStr=Enum: enmBmsFaultLvl
  Data Type Conversion : DataTypeConversion  OutDataTypeStr=uint8
  Detect Change : simulink/Logic and Bit Operations/Detect Change  vinit=0  OutDataTypeStr=boolean
  Logical Operator10 : Logic  Operator=OR  Inputs=3  AllPortsSameDT=off  OutDataTypeStr=boolean
  Relational Operator2 : RelationalOperator  OutDataTypeStr=boolean  RndMeth=Simplest
  BTMR_ThmEndCom : Outport
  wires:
  DSMR_stFaultRank/1 -> Relational Operator2/1
  Relational Operator2/1 -> Logical Operator10/2
  Constant13/1 -> Data Type Conversion/1
  Logical Operator10/1 -> BTMR_ThmEndCom/1
  COMR_bLeadAcidChgHvOn/1 -> Logical Operator10/3
  BMCR_stBmsModeCtrl/1 -> Detect Change/1
  Detect Change/1 -> Logical Operator10/1
  Data Type Conversion/1 -> Relational Operator2/2

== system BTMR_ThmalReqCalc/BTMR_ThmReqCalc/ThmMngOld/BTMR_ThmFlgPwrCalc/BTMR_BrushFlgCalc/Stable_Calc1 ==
  source_Uint : Inport
  cntStable : Inport  Port=2
  Chart : Stateflow chart  TreatAsAtomicUnit=on
  Delay1 : Delay  DelayLength=1  InitialCondition=0
  Detect Change : simulink/Logic and Bit Operations/Detect Change  vinit=0  OutDataTypeStr=boolean
  Switch : Switch  Criteria=u2 ~= 0
  stableOut : Outport
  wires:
  Detect Change/1 -> Chart/1(trigger_in)
  cntStable/1 -> Chart/2(cntStable)
  Chart/1(flg_out) -> Switch/2
  Delay1/1 -> Switch/1
  Switch/1 -> Delay1/1, stableOut/1
  source_Uint/1 -> Switch/3, Detect Change/1

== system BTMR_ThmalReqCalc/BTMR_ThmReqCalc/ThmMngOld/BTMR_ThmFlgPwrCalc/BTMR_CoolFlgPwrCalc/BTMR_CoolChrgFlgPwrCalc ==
  BTMR_flgCoolChrgTempSgns : Inport
  Enable : EnablePort  StatesWhenEnabling=reset
  BSER_ClntPwrReqCalc : Subsystem
  BSER_ClntPwrReqFlgCalc : Subsystem
  Bus Selector : BusSelector  OutputSignals=BTMR_flgCoolChrgInTempSgns,BTMR_flgCoolChrgIntTempSgns
  Bus Selector1 : BusSelector  OutputSignals=BTMR_flgCoolChrgStage2EnaTemp,BTMR_flgCoolChrgStage3EnaTemp,BTMR_flgCoolChrgStage2ExtTemp,BTMR_flgCoolChrgStage3ExtTemp
  Bus Selector2 : BusSelector  OutputSignals=BTMR_flgCoolChrgStage1PowRedTemp,BTMR_flgCoolChrgStage1PowResTemp,BTMR_flgCoolChrgStage2PowRedTemp,BTMR_flgCoolChrgStage2PowResTemp,BTMR_flgCoolChrgStage3PowRedTemp,BTMR_flgCoolChrgStage3PowResTemp
  Chart : Stateflow chart  TreatAsAtomicUnit=on
  Constant12 : Constant  Value=BTMR_cntThmalReqVal_C
  Data Type Conversion : DataTypeConversion  OutDataTypeStr=uint8
  Stable_Calc : Subsystem
  BTMR_flgClntPwrReq : Outport  InitialOutput=0
  BTMR_pClntPwrReq : Outport  Port=2  InitialOutput=0
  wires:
  BTMR_flgCoolChrgTempSgns/1 -> Bus Selector/1
  Bus Selector/1 -> Bus Selector1/1  "<BTMR_flgCoolChrgInTempSgns>"
  Bus Selector/2 -> Bus Selector2/1  "<BTMR_flgCoolChrgIntTempSgns>"
  Bus Selector1/1 -> Chart/1(CoolChrgStage2Ena)  "<BTMR_flgCoolChrgStage2EnaTemp>"
  Bus Selector1/2 -> Chart/2(CoolChrgStage3Ena)  "<BTMR_flgCoolChrgStage3EnaTemp>"
  Bus Selector1/3 -> Chart/3(CoolChrgStage2Ext)  "<BTMR_flgCoolChrgStage2ExtTemp>"
  Bus Selector1/4 -> Chart/4(CoolChrgStage3Ext)  "<BTMR_flgCoolChrgStage3ExtTemp>"
  Bus Selector2/1 -> Chart/5(CoolChrgStage1PowRed)  "<BTMR_flgCoolChrgStage1PowRedTemp>"
  Bus Selector2/2 -> Chart/6(CoolChrgStage1PowRes)  "<BTMR_flgCoolChrgStage1PowResTemp>"
  Bus Selector2/3 -> Chart/7(CoolChrgStage2PowRed)  "<BTMR_flgCoolChrgStage2PowRedTemp>"
  Bus Selector2/4 -> Chart/8(CoolChrgStage2PowRes)  "<BTMR_flgCoolChrgStage2PowResTemp>"
  Bus Selector2/5 -> Chart/9(CoolChrgStage3PowRed)  "<BTMR_flgCoolChrgStage3PowRedTemp>"
  Bus Selector2/6 -> Chart/10(CoolChrgStage3PowRes)  "<BTMR_flgCoolChrgStage3PowResTemp>"
  Stable_Calc/1(stableOut) -> BSER_ClntPwrReqCalc/1(BTMR_stsClntStg), BSER_ClntPwrReqFlgCalc/1(BTMR_stsClntStg)
  Chart/1(BTMR_stsClntStg) -> Data Type Conversion/1
  BSER_ClntPwrReqFlgCalc/1(BTMR_flgClntPwrReq) -> BTMR_flgClntPwrReq/1
  BSER_ClntPwrReqCalc/1(BTMR_pClntPwrReq) -> BTMR_pClntPwrReq/1
  Constant12/1 -> Stable_Calc/2(cntStable)
  Data Type Conversion/1 -> Stable_Calc/1(source_Uint)

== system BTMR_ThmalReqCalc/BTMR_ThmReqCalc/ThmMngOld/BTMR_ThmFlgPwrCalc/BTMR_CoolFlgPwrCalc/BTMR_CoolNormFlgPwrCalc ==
  BTMR_flgCoolNormTempSgns : Inport
  Enable : EnablePort  StatesWhenEnabling=reset
  BSER_ClntPwrReqCalc : Subsystem
  BSER_ClntPwrReqFlgCalc : Subsystem
  Bus Selector : BusSelector  OutputSignals=BTMR_flgCoolNormInTempSgns,BTMR_flgCoolNormIntTempSgns
  Bus Selector1 : BusSelector  OutputSignals=BTMR_flgCoolNormStage2EnaTemp,BTMR_flgCoolNormStage3EnaTemp,BTMR_flgCoolNormStage2ExtTemp,BTMR_flgCoolNormStage3ExtTemp
  Bus Selector2 : BusSelector  OutputSignals=BTMR_flgCoolNormPowRedTemp,BTMR_flgCoolNormPowResTemp
  Chart : Stateflow chart  TreatAsAtomicUnit=on
  Constant12 : Constant  Value=BTMR_cntThmalReqVal_C
  Data Type Conversion : DataTypeConversion  OutDataTypeStr=uint8
  Stable_Calc : Subsystem
  BTMR_flgClntPwrReq : Outport  InitialOutput=0
  BTMR_pClntPwrReq : Outport  Port=2  InitialOutput=0
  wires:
  BTMR_flgCoolNormTempSgns/1 -> Bus Selector/1
  Bus Selector/1 -> Bus Selector1/1  "<BTMR_flgCoolNormInTempSgns>"
  Bus Selector/2 -> Bus Selector2/1  "<BTMR_flgCoolNormIntTempSgns>"
  Bus Selector1/1 -> Chart/1(CoolNormStage2Ena)  "<BTMR_flgCoolNormStage2EnaTemp>"
  Bus Selector1/2 -> Chart/2(CoolNormStage3Ena)  "<BTMR_flgCoolNormStage3EnaTemp>"
  Bus Selector1/3 -> Chart/3(CoolNormStage2Ext)  "<BTMR_flgCoolNormStage2ExtTemp>"
  Bus Selector1/4 -> Chart/4(CoolNormStage3Ext)  "<BTMR_flgCoolNormStage3ExtTemp>"
  Bus Selector2/1 -> Chart/5(CoolNormPowRed)  "<BTMR_flgCoolNormPowRedTemp>"
  Bus Selector2/2 -> Chart/6(CoolNormPowRes)  "<BTMR_flgCoolNormPowResTemp>"
  Chart/1(BTMR_stsClntStg) -> Data Type Conversion/1
  Stable_Calc/1(stableOut) -> BSER_ClntPwrReqCalc/1(BTMR_stsClntStg), BSER_ClntPwrReqFlgCalc/1(BTMR_stsClntStg)
  BSER_ClntPwrReqFlgCalc/1(BTMR_flgClntPwrReq) -> BTMR_flgClntPwrReq/1
  BSER_ClntPwrReqCalc/1(BTMR_pClntPwrReq) -> BTMR_pClntPwrReq/1
  Constant12/1 -> Stable_Calc/2(cntStable)
  Data Type Conversion/1 -> Stable_Calc/1(source_Uint)

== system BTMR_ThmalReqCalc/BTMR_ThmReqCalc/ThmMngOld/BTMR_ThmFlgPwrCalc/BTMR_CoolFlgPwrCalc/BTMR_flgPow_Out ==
  stCoolSts : Inport
  BTMR_flgBrsPwrReq : Inport  Port=2
  BTMR_flgClntPwrReqMerge : Inport  Port=3
  BTMR_pClntPwrReqMerge : Inport  Port=4
  Constant1 : Constant  Value=BTMR_pCoolPwrVal_C
  Constant16 : Constant  Value=single(0)
  Constant2 : Constant  Value=BTMR_flgCoolPwrCal_C
  Constant4 : Constant  Value=single(0)
  Constant5 : Constant  Value=enmThmCoolFlg.FLASH  OutDataTypeStr=Enum: enmThmCoolFlg
  Constant7 : Constant  Value=enmThmCoolFlg.INACTIVE  OutDataTypeStr=Enum: enmThmCoolFlg
  Conversion1 : DataTypeConversion  OutDataTypeStr=uint8
  Data Type Conversion2 : DataTypeConversion  OutDataTypeStr=uint8
  Data Type Conversion5 : DataTypeConversion  OutDataTypeStr=uint8
  Switch{1..4,8,11} (6 alike) : Switch  Criteria=u2 ~= 0
  BTMR_flgClntPwrReq : Outport
  BTMR_pClntPwrReq : Outport  Port=2
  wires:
  Constant5/1 -> Data Type Conversion2/1
  Data Type Conversion2/1 -> Switch2/1
  Constant2/1 -> Switch8/2, Conversion1/1, Switch1/2
  Switch3/1 -> Switch8/3
  Switch4/1 -> Switch2/3, Switch11/2
  Constant4/1 -> Switch3/1
  Constant1/1 -> Switch8/1
  Switch2/1 -> Switch1/3
  BTMR_flgBrsPwrReq/1 -> Switch3/2, Switch2/2
  Switch11/1 -> Switch3/3
  Conversion1/1 -> Switch1/1
  Switch8/1 -> BTMR_pClntPwrReq/1
  Switch1/1 -> BTMR_flgClntPwrReq/1
  Constant7/1 -> Data Type Conversion5/1
  BTMR_flgClntPwrReqMerge/1 -> Switch4/1
  Data Type Conversion5/1 -> Switch4/3
  Constant16/1 -> Switch11/3
  BTMR_pClntPwrReqMerge/1 -> Switch11/1
  stCoolSts/1 -> Switch4/2

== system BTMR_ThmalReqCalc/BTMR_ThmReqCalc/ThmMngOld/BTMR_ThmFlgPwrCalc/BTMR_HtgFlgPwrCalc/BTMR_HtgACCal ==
  Enable : EnablePort  StatesWhenEnabling=reset
  Constant2 : Constant  Value=enmThmHeatFlg.ACTIVE  OutDataTypeStr=Enum: enmThmHeatFlg
  Constant3 : Constant  Value=BTMR_pHtgACPwrReq_C
  Data Type Conversion1 : DataTypeConversion  OutDataTypeStr=uint8
  BTMR_flgHtgPwrReq : Outport  InitialOutput=0
  BTMR_pHtgPwrReq : Outport  Port=2  InitialOutput=0
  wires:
  Constant3/1 -> BTMR_pHtgPwrReq/1
  Data Type Conversion1/1 -> BTMR_flgHtgPwrReq/1
  Constant2/1 -> Data Type Conversion1/1

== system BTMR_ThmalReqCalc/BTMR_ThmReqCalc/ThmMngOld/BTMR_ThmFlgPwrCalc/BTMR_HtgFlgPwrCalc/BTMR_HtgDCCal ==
  BTMR_flgHtgDCCalSgns : Inport
  BTMR_pHtgDCPowCur : Inport  Port=2
  Enable : EnablePort  StatesWhenEnabling=reset
  BSER_HeatPwrReqCalc : Subsystem
  BSER_HeatPwrReqFlgCalc : Subsystem
  Bus Selector : BusSelector  OutputSignals=BTMR_flgHtgDCTempSgns
  Bus Selector1 : BusSelector  OutputSignals=BTMR_pHtgDCPowCur1,BTMR_pHtgDCPowCur2
  Bus Selector2 : BusSelector  OutputSignals=BTMR_flgHtgDCIntTempSgns
  Bus Selector4 : BusSelector  OutputSignals=BTMR_flgHtgDCStage2EnaTemp,BTMR_HtgDCStage2PowRedTemp,BTMR_HtgDCStage2PowResTemp,BTMR_HtgDCStage3PowRedTemp
  Chart : Stateflow chart  TreatAsAtomicUnit=on
  Constant12 : Constant  Value=BTMR_cntThmalReqVal_C
  Data Type Conversion : DataTypeConversion  OutDataTypeStr=uint8
  Stable_Calc : Subsystem
  BTMR_flgHtgPwrReq : Outport  InitialOutput=0
  BTMR_pHtgPwrReq : Outport  Port=2  InitialOutput=0
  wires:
  BTMR_pHtgDCPowCur/1 -> Bus Selector1/1
  BTMR_flgHtgDCCalSgns/1 -> Bus Selector/1
  Bus Selector1/1 -> BSER_HeatPwrReqCalc/2(HtgDCPowCur1)  "<BTMR_pHtgDCPowCur1>"
  Bus Selector1/2 -> BSER_HeatPwrReqCalc/3(HtgDCPowCur2)  "<BTMR_pHtgDCPowCur2>"
  Bus Selector/1 -> Bus Selector2/1  "<BTMR_flgHtgDCTempSgns>"
  Bus Selector2/1 -> Bus Selector4/1  "<BTMR_flgHtgDCIntTempSgns>"
  Bus Selector4/1 -> Chart/1(HtgDCStage2Ena)  "<BTMR_flgHtgDCStage2EnaTemp>"
  Bus Selector4/2 -> Chart/2(HtgDCStage2PowRed)  "<BTMR_HtgDCStage2PowRedTemp>"
  Bus Selector4/3 -> Chart/3(HtgDCStage2PowRes)  "<BTMR_HtgDCStage2PowResTemp>"
  Bus Selector4/4 -> Chart/4(HtgDCStage3PowRed)  "<BTMR_HtgDCStage3PowRedTemp>"
  Stable_Calc/1(stableOut) -> BSER_HeatPwrReqCalc/1(BTMR_stsHeatStg), BSER_HeatPwrReqFlgCalc/1(BTMR_stsHeatStg)
  Chart/1(BTMR_stsHeatStg) -> Data Type Conversion/1
  BSER_HeatPwrReqCalc/1(BTMR_pHtgPwrReq) -> BTMR_pHtgPwrReq/1
  BSER_HeatPwrReqFlgCalc/1(BTMR_flgHtgPwrReq) -> BTMR_flgHtgPwrReq/1
  Constant12/1 -> Stable_Calc/2(cntStable)
  Data Type Conversion/1 -> Stable_Calc/1(source_Uint)

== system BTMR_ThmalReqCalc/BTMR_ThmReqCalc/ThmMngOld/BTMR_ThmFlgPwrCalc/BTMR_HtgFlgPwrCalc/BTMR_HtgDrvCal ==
  Enable : EnablePort  StatesWhenEnabling=reset
  Constant1 : Constant  Value=BTMR_pHtgDrvPwrReq_C
  Constant2 : Constant  Value=enmThmHeatFlg.ACTIVE  OutDataTypeStr=Enum: enmThmHeatFlg
  Data Type Conversion1 : DataTypeConversion  OutDataTypeStr=uint8
  BTMR_flgHtgPwrReq : Outport  InitialOutput=0
  BTMR_pHtgPwrReq : Outport  Port=2  InitialOutput=0
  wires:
  Constant2/1 -> Data Type Conversion1/1
  Data Type Conversion1/1 -> BTMR_flgHtgPwrReq/1
  Constant1/1 -> BTMR_pHtgPwrReq/1

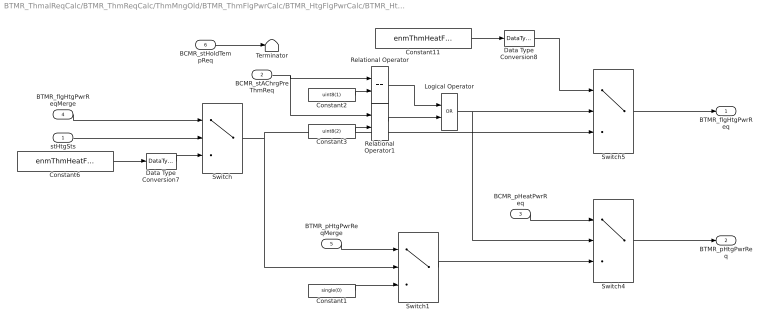
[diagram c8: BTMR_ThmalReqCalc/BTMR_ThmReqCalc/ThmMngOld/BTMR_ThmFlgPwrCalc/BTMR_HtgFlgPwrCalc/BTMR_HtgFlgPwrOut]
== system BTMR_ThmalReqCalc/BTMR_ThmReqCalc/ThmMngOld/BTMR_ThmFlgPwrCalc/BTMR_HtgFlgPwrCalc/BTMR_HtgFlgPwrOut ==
  stHtgSts : Inport
  BCMR_stAChrgPreThmReq : Inport  Port=2
  BCMR_pHeatPwrReq : Inport  Port=3
  BTMR_flgHtgPwrReqMerge : Inport  Port=4
  BTMR_pHtgPwrReqMerge : Inport  Port=5
  BCMR_stHoldTempReq : Inport  Port=6
  Constant1 : Constant  Value=single(0)
  Constant11 : Constant  Value=enmThmHeatFlg.INACTIVE  OutDataTypeStr=Enum: enmThmHeatFlg
  Constant2 : Constant  Value=uint8(1)
  Constant3 : Constant  Value=uint8(2)
  Constant6 : Constant  Value=enmThmHeatFlg.INACTIVE  OutDataTypeStr=Enum: enmThmHeatFlg
  Data Type Conversion7 : DataTypeConversion  OutDataTypeStr=uint8
  Data Type Conversion8 : DataTypeConversion  OutDataTypeStr=uint8
  Logical Operator : Logic  Operator=OR  AllPortsSameDT=off  OutDataTypeStr=boolean
  Relational Operator : RelationalOperator  Operator===  OutDataTypeStr=boolean  RndMeth=Simplest
  Relational Operator1 : RelationalOperator  Operator===  OutDataTypeStr=boolean  RndMeth=Simplest
  Switch{,1,4..5} (4 alike) : Switch  Criteria=u2 ~= 0
  Terminator : Terminator
  BTMR_flgHtgPwrReq : Outport
  BTMR_pHtgPwrReq : Outport  Port=2
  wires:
  Switch1/1 -> Switch4/3
  BTMR_pHtgPwrReqMerge/1 -> Switch1/1
  stHtgSts/1 -> Switch/2
  Constant1/1 -> Switch1/3
  Logical Operator/1 -> Switch4/2, Switch5/2
  BCMR_pHeatPwrReq/1 -> Switch4/1
  Constant11/1 -> Data Type Conversion8/1
  Switch/1 -> Switch5/3, Switch1/2
  Switch4/1 -> BTMR_pHtgPwrReq/1
  BTMR_flgHtgPwrReqMerge/1 -> Switch/1
  Data Type Conversion8/1 -> Switch5/1
  Switch5/1 -> BTMR_flgHtgPwrReq/1
  Data Type Conversion7/1 -> Switch/3
  Constant6/1 -> Data Type Conversion7/1
  BCMR_stHoldTempReq/1 -> Terminator/1
  BCMR_stAChrgPreThmReq/1 -> Relational Operator1/1, Relational Operator/1
  Relational Operator/1 -> Logical Operator/1
  Constant2/1 -> Relational Operator/2
  Constant3/1 -> Relational Operator1/2
  Relational Operator1/1 -> Logical Operator/2

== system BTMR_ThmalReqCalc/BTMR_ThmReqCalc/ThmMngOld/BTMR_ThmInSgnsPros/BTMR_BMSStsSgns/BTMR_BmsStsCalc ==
  BMCR_stBmsModeCtrl : Inport
  COMR_bLeadAcidChgHvOn : Inport  Port=2
  Bus Creator : BusCreator  Inputs=4
  Data Type Conversion : DataTypeConversion  OutDataTypeStr=uint8
  Data Type Conversion1 : DataTypeConversion  OutDataTypeStr=uint8
  Data Type Conversion2 : DataTypeConversion  OutDataTypeStr=uint8
  Logical Operator1 : Logic  Operator=NOT  Inputs=3  AllPortsSameDT=off  OutDataTypeStr=boolean
  Logical Operator10 : Logic  Operator=OR  Inputs=3  AllPortsSameDT=off  OutDataTypeStr=boolean
  Logical Operator2 : Logic  AllPortsSameDT=off  OutDataTypeStr=boolean
  Logical Operator3 : Logic  Operator=NOT  AllPortsSameDT=off  OutDataTypeStr=boolean
  Relational Operator3 : RelationalOperator  Operator===  OutDataTypeStr=boolean  RndMeth=Simplest
  Relational Operator4 : RelationalOperator  Operator===  OutDataTypeStr=boolean  RndMeth=Simplest
  Relational Operator5 : RelationalOperator  Operator===  OutDataTypeStr=boolean  RndMeth=Simplest
  stBms_DChrg : Constant  Value=enmThmBmsSts.DCChrg  OutDataTypeStr=Enum: enmThmBmsSts
  stBms_DChrg1 : Constant  Value=enmThmBmsSts.ACChrg  OutDataTypeStr=Enum: enmThmBmsSts
  stBms_DChrg2 : Constant  Value=enmThmBmsSts.HvOn  OutDataTypeStr=Enum: enmThmBmsSts
  BTMR_flgBMSSgns : Outport
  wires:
  Data Type Conversion2/1 -> Relational Operator5/2
  BMCR_stBmsModeCtrl/1 -> Relational Operator3/1, Relational Operator4/1, Relational Operator5/1
  stBms_DChrg/1 -> Data Type Conversion/1
  Data Type Conversion1/1 -> Relational Operator4/2
  Logical Operator2/1 -> Bus Creator/3, Logical Operator10/3  "BTMR_flgBMSDrv"
  Relational Operator3/1 -> Bus Creator/1, Logical Operator10/1  "BTMR_flgBMSDChrg"
  Relational Operator4/1 -> Bus Creator/2, Logical Operator10/2  "BTMR_flgBMSAChrg"
  Logical Operator10/1 -> Logical Operator1/1
  Bus Creator/1 -> BTMR_flgBMSSgns/1
  Logical Operator1/1 -> Bus Creator/4  "BTMR_flgBMSOther"
  Relational Operator5/1 -> Logical Operator2/1  "BTMR_flgBMSHV"
  COMR_bLeadAcidChgHvOn/1 -> Logical Operator3/1
  Logical Operator3/1 -> Logical Operator2/2
  Data Type Conversion/1 -> Relational Operator3/2
  stBms_DChrg1/1 -> Data Type Conversion1/1
  stBms_DChrg2/1 -> Data Type Conversion2/1

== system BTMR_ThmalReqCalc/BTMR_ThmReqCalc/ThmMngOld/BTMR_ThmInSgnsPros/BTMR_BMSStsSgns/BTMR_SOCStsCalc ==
  BSER_rSoc : Inport
  Bus Creator1 : BusCreator  Inputs=2
  Constant18 : Constant  Value=BTMR_r861HtgDrvSoc_C
  Constant21 : Constant  Value=BTMR_r861BrsDrvSoc_C
  Relational Operator6 : RelationalOperator  Operator=>  OutDataTypeStr=boolean  RndMeth=Simplest
  Relational Operator7 : RelationalOperator  Operator=>  OutDataTypeStr=boolean  RndMeth=Simplest
  BTMR_flgSOCSgns : Outport
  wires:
  Constant18/1 -> Relational Operator6/2
  BSER_rSoc/1 -> Relational Operator6/1, Relational Operator7/1
  Constant21/1 -> Relational Operator7/2
  Relational Operator7/1 -> Bus Creator1/1  "BTMR_flgBrsDrvSOC"
  Relational Operator6/1 -> Bus Creator1/2  "BTMR_flgHtgDrvSOC"
  Bus Creator1/1 -> BTMR_flgSOCSgns/1

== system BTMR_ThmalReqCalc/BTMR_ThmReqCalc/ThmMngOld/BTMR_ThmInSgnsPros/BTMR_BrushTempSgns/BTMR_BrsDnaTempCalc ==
  BSPR_tCellTempMin : Inport
  BSPR_tCellTempMax : Inport  Port=2
  Add : Sum  Inputs=+-
  Add1 : Sum  Inputs=+-
  BMSDebounceStartZero : AIWAYS_Powertrain_BMS_lib/Debounce & Delay/BMSDebounceStartZero
  Constant2 : Constant  Value=BTMR_t861BrsDiffLv0Temp_C
  Constant29 : Constant  Value=BTMR_tiTempBase_C
  Constant30 : Constant  Value=BTMR_tiTempDebs_C
  Constant4 : Constant  Value=BTMR_tBrsMinCellTempThre_C
  Constant5 : Constant  Value=BTMR_tBrsMinCellTempDeb_C
  Logical Operator2 : Logic  Operator=OR  AllPortsSameDT=off  OutDataTypeStr=boolean
  Relational Operator1 : RelationalOperator  Operator=<=  OutDataTypeStr=boolean  RndMeth=Simplest
  Relational Operator2 : RelationalOperator  Operator=<=  OutDataTypeStr=boolean  RndMeth=Simplest
  BTMR_flgBrsDnaTemp : Outport
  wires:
  BSPR_tCellTempMax/1 -> Add/1
  Logical Operator2/1 -> BMSDebounceStartZero/1
  Constant2/1 -> Relational Operator2/2
  Add/1 -> Relational Operator2/1
  BMSDebounceStartZero/1 -> BTMR_flgBrsDnaTemp/1
  Constant29/1 -> BMSDebounceStartZero/5, BMSDebounceStartZero/3
  Constant30/1 -> BMSDebounceStartZero/4, BMSDebounceStartZero/2
  Constant4/1 -> Add1/1
  Constant5/1 -> Add1/2
  Add1/1 -> Relational Operator1/2
  BSPR_tCellTempMin/1 -> Relational Operator1/1, Add/2
  Relational Operator2/1 -> Logical Operator2/1
  Relational Operator1/1 -> Logical Operator2/2
